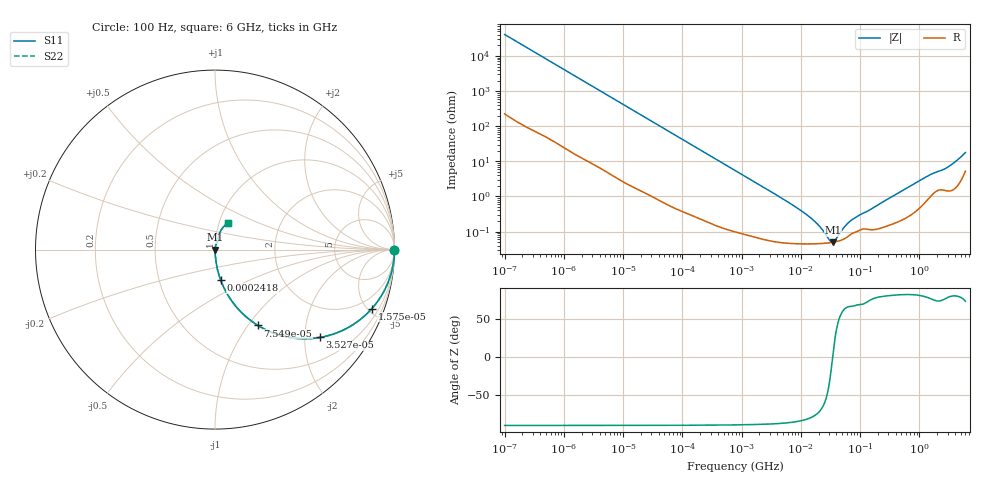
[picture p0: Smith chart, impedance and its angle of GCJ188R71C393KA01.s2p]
!Murata Part Number: GCJ188R71C393KA01
!These Parameters are Measured in Series Mode Connection
!Data Generated on Mar 13, 2026
!  o--ll--o
!Port1  Port2
!  o------o
!Operation Temp=25[degC], DC Bias Voltage=0[V]
!Freq. Start=100[Hz] Stop=6[GHz] 401[Steps]
# Hz S RI R 50
!Freq.(Hz) S11(Real) S11(Imag) S21(Real) S21(Imag) S12(Real) S12(Imag) S22(Real) S22(Imag)
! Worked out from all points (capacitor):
!   401 points, 100 Hz to 6 GHz, reference 50 ohm
!   read as one part in series: C = 38.7 nF near 109 Hz
!   lowest |Z| = 49.5 mohm at 34.83 MHz (marker M1)
!   series resonance near 34.48 MHz, so ESL is about 550 pH
!   S11 on the Smith chart (normalised r, x): 100 Hz: open; 15.75 kHz: 1.03, -5.31; 35.27 kHz: 1.02, -2.38; 75.5 kHz: 1.01, -1.11; 241.8 kHz: 1.00, -0.35; 6 GHz: 1.10, +0.34
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100  1 -0.00244  1.92e-05 0.00244  1.92e-05 0.00244  1 -0.00244
2008  0.9974 -0.0483  0.00263 0.0483  0.00263 0.0483  0.9974 -0.0483
6151  0.9778 -0.1442  0.0222 0.1442  0.0222 0.1442  0.9778 -0.1442
15752  0.8741 -0.3285  0.1259 0.3285  0.1259 0.3285  0.8741 -0.3285
35265  0.5854 -0.489  0.4146 0.489  0.4146 0.489  0.5854 -0.489
40335  0.5198 -0.4959  0.4802 0.4959  0.4802 0.4959  0.5198 -0.4959
75495  0.2389 -0.4224  0.7611 0.4224  0.7611 0.4224  0.2389 -0.4224
129199  0.0986 -0.2935  0.9014 0.2935  0.9014 0.2935  0.0986 -0.2935
241822  0.0316 -0.1693  0.9684 0.1693  0.9684 0.1693  0.0316 -0.1693
774597  0.00399 -0.0547  0.996 0.0547  0.996 0.0547  0.00399 -0.0547
6353432  0.000503 -0.00657  0.9995 0.00657  0.9995 0.00657  0.000503 -0.00657
1.555665e7  0.00045 -0.00221  0.9995 0.00221  0.9995 0.00221  0.00045 -0.00221
2.128304e7  0.000455 -0.00126  0.9995 0.00126  0.9995 0.00126  0.000455 -0.00126
3.045065e7  0.000478 -0.000313  0.9995 0.000313  0.9995 0.000313  0.000478 -0.000313
3.482834e7  0.000494 2.57e-05  0.9995 -2.57e-05  0.9995 -2.57e-05  0.000494 2.57e-05
3.80911e7  0.000508 0.000252  0.9995 -0.000252  0.9995 -0.000252  0.000508 0.000252
5.699437e7  0.000651 0.00132  0.9993 -0.00132  0.9993 -0.00132  0.000651 0.00132
7.129496e7  0.000854 0.00192  0.9991 -0.00192  0.9991 -0.00192  0.000854 0.00192
3.124326e8  0.00159 0.00878  0.9984 -0.00878  0.9984 -0.00878  0.00159 0.00878
1.369159e9  0.00918 0.0362  0.9908 -0.0362  0.9908 -0.0362  0.00918 0.0362
2.931063e9  0.0182 0.0624  0.9818 -0.0624  0.9818 -0.0624  0.0182 0.0624
6e9  0.0739 0.1496  0.9261 -0.1496  0.9261 -0.1496  0.0739 0.1496
